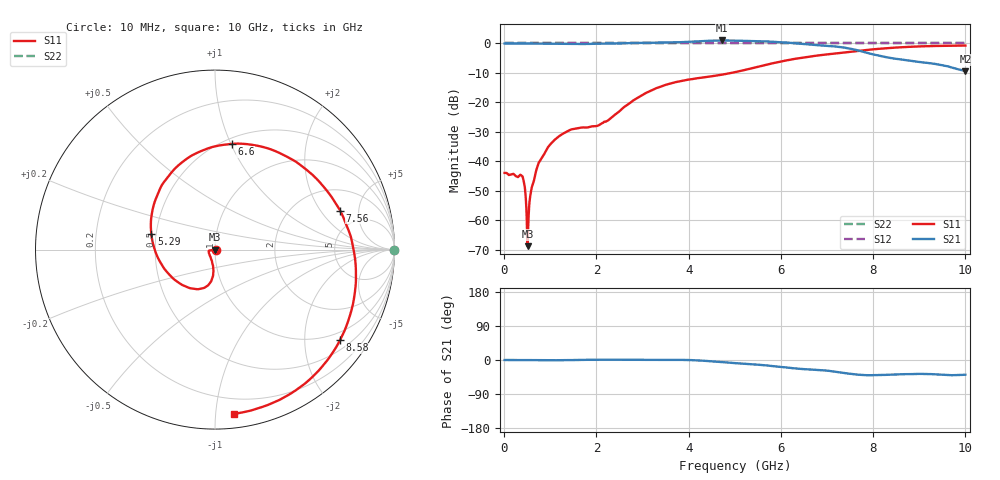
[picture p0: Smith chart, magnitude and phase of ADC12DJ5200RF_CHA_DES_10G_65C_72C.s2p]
! Texas Instruments, Inc.
! ADC12DJ5200RF - CH A S-Parameters (DES Mode, Fs = 10 GSPS, 65 degC case, 72 degC juntion)
! Port 1 represents the 100-ohm differenal input, Port 2 the digital output
! freq  dbS11  angS11  dbS21 angS21 dbS12 angS12 dbS22 angS22
# HZ S DB R 100
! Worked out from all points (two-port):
!   1000 points, 10 MHz to 10 GHz, reference 100 ohm
!   highest |S21| = 1.02 dB at 4.73 GHz (marker M1); lowest = -9.4 dB at 10 GHz (marker M2)
!   |S21| within 3 dB of the highest: start of sweep to 7.569 GHz
!   lowest |S11| = -68.9 dB at 510 MHz (marker M3), VSWR 1.00, Z = 100 - j0.0713 ohm
!   |S11| at or under -10 dB: start of sweep to 4.932 GHz
!   |S22| runs from 0.0 to 0.0 dB; largest |S21 - S12| = 0.77
!   S11 on the Smith chart (normalised r, x): 10 MHz: 1.01, -0.00; 5.29 GHz: 0.47, +0.10; 6.6 GHz: 0.55, +1.01; 7.56 GHz: 3.35, +3.13; 8.58 GHz: 0.75, -2.91; 10 GHz: 0.09, -1.12
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1e7  -43.98 -7.6  0.00 -0.0  0.00 0.0  0.00 0.0
3.8e8  -44.92 -10.5  0.00 -0.4  0.00 0.0  0.00 0.0
4.3e8  -47.24 -0.5  -0.01 -0.5  0.00 0.0  0.00 0.0
4.7e8  -52.81 6.8  -0.01 -0.5  0.00 0.0  0.00 0.0
5.1e8  -68.87 -81.6  -0.02 -0.5  0.00 0.0  0.00 0.0
6e8  -48.82 -136.8  -0.02 -0.6  0.00 0.0  0.00 0.0
7.1e8  -42.37 -157.4  -0.06 -0.5  0.00 0.0  0.00 0.0
9.4e8  -35.52 -169.1  -0.07 -0.6  0.00 0.0  0.00 0.0
1.26e9  -30.80 -171.7  -0.15 -0.6  0.00 0.0  0.00 0.0
1.68e9  -28.56 -163.4  -0.19 0.3  0.00 0.0  0.00 0.0
2.24e9  -26.25 -119.8  -0.02 0.7  0.00 0.0  0.00 0.0
3.34e9  -14.98 -96.9  0.26 0.3  0.00 0.0  0.00 0.0
4.73e9  -10.59 -155.1  1.02 -5.6  0.00 0.0  0.00 0.0
5.01e9  -9.74 -174.4  0.96 -8.3  0.00 0.0  0.00 0.0
5.29e9  -8.74 165.9  0.82 -10.5  0.00 0.0  0.00 0.0
5.9e9  -6.49 126.2  0.53 -17.1  0.00 0.0  0.00 0.0
6.6e9  -4.49 81.1  -0.35 -24.7  0.00 0.0  0.00 0.0
6.67e9  -4.33 76.5  -0.46 -25.3  0.00 0.0  0.00 0.0
7.56e9  -2.73 17.4  -1.95 -37.3  0.00 0.0  0.00 0.0
8.34e9  -1.56 -25.8  -4.83 -38.9  0.00 0.0  0.00 0.0
8.58e9  -1.31 -35.9  -5.38 -37.6  0.00 0.0  0.00 0.0
1e10  -0.71 -83.2  -9.41 -38.8  0.00 0.0  0.00 0.0
